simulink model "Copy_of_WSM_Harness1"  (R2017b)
settings: Solver=FixedStepDiscrete  StartTime=0.0  StopTime=2  FixedStep=0.01  RelTol=1e-3  EnableMultiTasking=on
undefined symbols (not defined in the file): sigbuilder_block

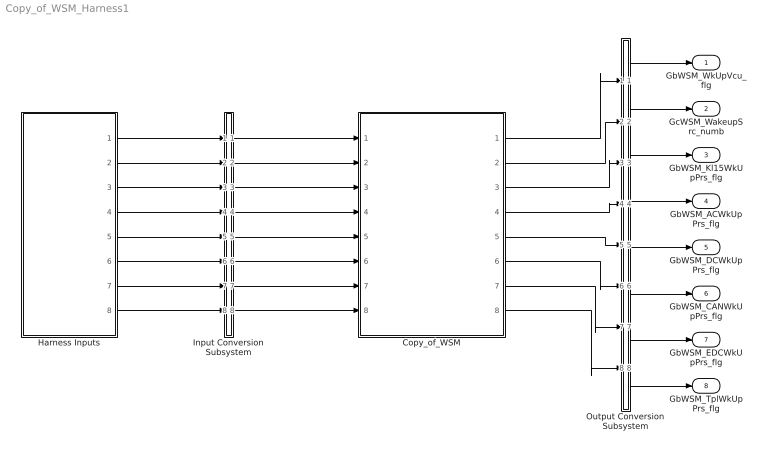
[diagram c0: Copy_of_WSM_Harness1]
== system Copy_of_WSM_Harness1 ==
  Copy_of_WSM : ModelReference  ModelNameDialog=Copy_of_WSM  SimulationMode=Normal  ModelReferenceVersion='M105C102'
  Harness Inputs : Subsystem  Tag=STV Subsys  LoadFcn=sigbuilder_block('load');  StartFcn=sigbuilder_block('start');  StopFcn=sigbuilder_block('stop');  ClipboardFcn=sigbuilder_block('clipboard');  mask(Sigbuilder block){tuvar=[0:10]}
      mask init:
      | if ~strcmp(get_param(bdroot(gcb),'SimulationStatus'),'stopped'),tuvar = sigbuilder_block('maskInit'); end
  Input Conversion Subsystem : Subsystem  Tag=__SLT_ICS__  Description=Signal spec. and routing
  Output Conversion Subsystem : Subsystem  Tag=__SLT_OCS__  Description=Signal spec. and routing
  GbWSM_WkUpVcu_flg : Outport  OutDataTypeStr=boolean  PortDimensions=[1]
  GcWSM_WakeupSrc_numb : Outport  Port=2  OutDataTypeStr=uint16  PortDimensions=[1]
  GbWSM_Kl15WkUpPrs_flg : Outport  Port=3  OutDataTypeStr=boolean  PortDimensions=[1]
  GbWSM_ACWkUpPrs_flg : Outport  Port=4  OutDataTypeStr=boolean  PortDimensions=[1]
  GbWSM_DCWkUpPrs_flg : Outport  Port=5  OutDataTypeStr=boolean  PortDimensions=[1]
  GbWSM_CANWkUpPrs_flg : Outport  Port=6  OutDataTypeStr=boolean  PortDimensions=[1]
  GbWSM_EDCWkUpPrs_flg : Outport  Port=7  OutDataTypeStr=boolean  PortDimensions=[1]
  GbWSM_TplWkUpPrs_flg : Outport  Port=8  OutDataTypeStr=boolean  PortDimensions=[1]
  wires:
  Harness Inputs/1(GbISP_Kl15WkUp_flg) -> Input Conversion Subsystem/1(Inport_1)
  Harness Inputs/2(GbISP_ObcWkUp_flg) -> Input Conversion Subsystem/2(Inport_2)
  Harness Inputs/3(GbLDP_DC12VSply_flg) -> Input Conversion Subsystem/3(Inport_3)
  Harness Inputs/4(GeISP_NetWkUpSt_enum) -> Input Conversion Subsystem/4(Inport_4)
  Harness Inputs/5(GeODP_ObcCcSt_enum) -> Input Conversion Subsystem/5(Inport_5)
  Harness Inputs/6(GbODP_2EBTiout_flg) -> Input Conversion Subsystem/6(Inport_6)
  Harness Inputs/7(GbISP_TFThmRnwyfDet_flg) -> Input Conversion Subsystem/7(Inport_7)
  Harness Inputs/8(GbTRA_TPLRnwyChkFinish_flg) -> Input Conversion Subsystem/8(Inport_8)
  Output Conversion Subsystem/1(Outport_1) -> GbWSM_WkUpVcu_flg/1
  Output Conversion Subsystem/2(Outport_2) -> GcWSM_WakeupSrc_numb/1
  Output Conversion Subsystem/3(Outport_3) -> GbWSM_Kl15WkUpPrs_flg/1
  Output Conversion Subsystem/4(Outport_4) -> GbWSM_ACWkUpPrs_flg/1
  Output Conversion Subsystem/5(Outport_5) -> GbWSM_DCWkUpPrs_flg/1
  Output Conversion Subsystem/6(Outport_6) -> GbWSM_CANWkUpPrs_flg/1
  Output Conversion Subsystem/7(Outport_7) -> GbWSM_EDCWkUpPrs_flg/1
  Output Conversion Subsystem/8(Outport_8) -> GbWSM_TplWkUpPrs_flg/1
  Input Conversion Subsystem/1(Outport_1) -> Copy_of_WSM/1
  Input Conversion Subsystem/2(Outport_2) -> Copy_of_WSM/2
  Input Conversion Subsystem/3(Outport_3) -> Copy_of_WSM/3
  Input Conversion Subsystem/4(Outport_4) -> Copy_of_WSM/4
  Input Conversion Subsystem/5(Outport_5) -> Copy_of_WSM/5
  Input Conversion Subsystem/6(Outport_6) -> Copy_of_WSM/6
  Input Conversion Subsystem/7(Outport_7) -> Copy_of_WSM/7
  Input Conversion Subsystem/8(Outport_8) -> Copy_of_WSM/8
  Copy_of_WSM/1 -> Output Conversion Subsystem/1(Inport_1)
  Copy_of_WSM/2 -> Output Conversion Subsystem/2(Inport_2)
  Copy_of_WSM/3 -> Output Conversion Subsystem/3(Inport_3)
  Copy_of_WSM/4 -> Output Conversion Subsystem/4(Inport_4)
  Copy_of_WSM/5 -> Output Conversion Subsystem/5(Inport_5)
  Copy_of_WSM/6 -> Output Conversion Subsystem/6(Inport_6)
  Copy_of_WSM/7 -> Output Conversion Subsystem/7(Inport_7)
  Copy_of_WSM/8 -> Output Conversion Subsystem/8(Inport_8)

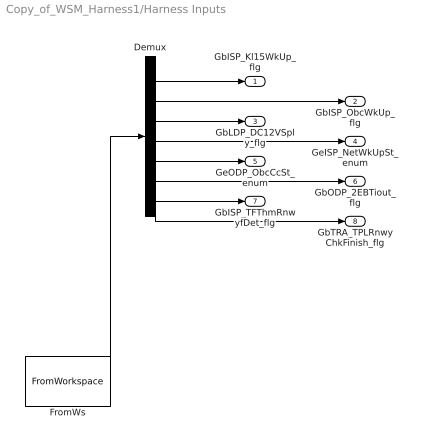
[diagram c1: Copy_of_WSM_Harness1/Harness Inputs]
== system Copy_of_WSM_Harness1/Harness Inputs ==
  Demux : Demux  Tag=STV Demux  Outputs=8
  FromWs : FromWorkspace  Tag=STV FromWs  VariableName=tuvar  SampleTime=0
  GbISP_Kl15WkUp_flg : Outport  Tag=STV Outport
  GbISP_ObcWkUp_flg : Outport  Tag=STV Outport  Port=2
  GbLDP_DC12VSply_flg : Outport  Tag=STV Outport  Port=3
  GeISP_NetWkUpSt_enum : Outport  Tag=STV Outport  Port=4
  GeODP_ObcCcSt_enum : Outport  Tag=STV Outport  Port=5
  GbODP_2EBTiout_flg : Outport  Tag=STV Outport  Port=6
  GbISP_TFThmRnwyfDet_flg : Outport  Tag=STV Outport  Port=7
  GbTRA_TPLRnwyChkFinish_flg : Outport  Tag=STV Outport  Port=8
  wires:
  FromWs/1 -> Demux/1
  Demux/1 -> GbISP_Kl15WkUp_flg/1
  Demux/2 -> GbISP_ObcWkUp_flg/1
  Demux/3 -> GbLDP_DC12VSply_flg/1
  Demux/4 -> GeISP_NetWkUpSt_enum/1
  Demux/5 -> GeODP_ObcCcSt_enum/1
  Demux/6 -> GbODP_2EBTiout_flg/1
  Demux/7 -> GbISP_TFThmRnwyfDet_flg/1
  Demux/8 -> GbTRA_TPLRnwyChkFinish_flg/1

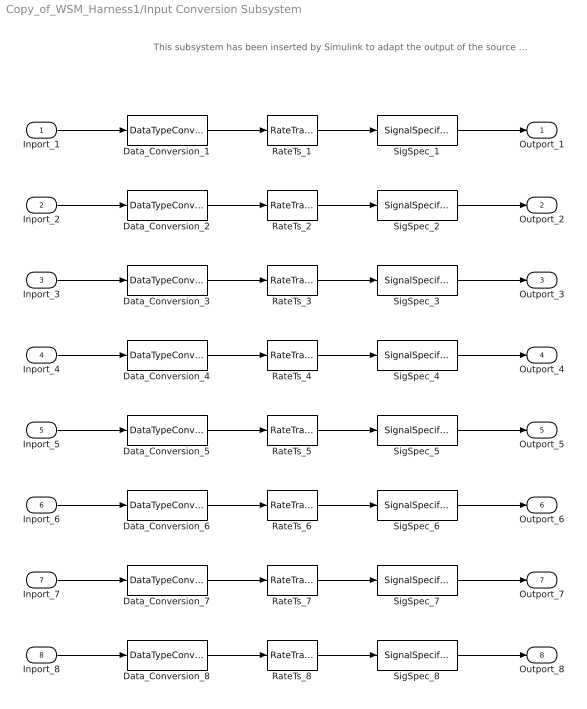
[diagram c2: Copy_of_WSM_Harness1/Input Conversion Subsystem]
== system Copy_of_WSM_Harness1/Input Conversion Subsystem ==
  note: This subsystem has been inserted by Simulink to adapt the output of the source blocks to the interface required by the harnessed component. Modifying the contents of this subsystem may result in compilation and simulation failure.
  Inport_1 : Inport
  Inport_2 : Inport  Port=2
  Inport_3 : Inport  Port=3
  Inport_4 : Inport  Port=4
  Inport_5 : Inport  Port=5
  Inport_6 : Inport  Port=6
  Inport_7 : Inport  Port=7
  Inport_8 : Inport  Port=8
  Data_Conversion_{1..3,6..8} (6 alike) : DataTypeConversion  OutDataTypeStr=boolean
  Data_Conversion_4 : DataTypeConversion  OutDataTypeStr=uint8
  Data_Conversion_5 : DataTypeConversion  OutDataTypeStr=uint8
  RateTs_{1..8} (8 alike) : RateTransition  OutPortSampleTime=0.01
  SigSpec_{1..3,7..8} (5 alike) : SignalSpecification  OutDataTypeStr=boolean  Unit=flag  Dimensions=[1]  SampleTime=0.01
  SigSpec_4 : SignalSpecification  OutDataTypeStr=uint8  Unit=enum  Dimensions=[1]  SampleTime=0.01
  SigSpec_5 : SignalSpecification  OutDataTypeStr=uint8  Unit=numb  Dimensions=[1]  SampleTime=0.01
  SigSpec_6 : SignalSpecification  OutDataTypeStr=boolean  Unit=flg  Dimensions=[1]  SampleTime=0.01
  Outport_1 : Outport
  Outport_2 : Outport  Port=2
  Outport_3 : Outport  Port=3
  Outport_4 : Outport  Port=4
  Outport_5 : Outport  Port=5
  Outport_6 : Outport  Port=6
  Outport_7 : Outport  Port=7
  Outport_8 : Outport  Port=8
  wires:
  SigSpec_1/1 -> Outport_1/1
  RateTs_1/1 -> SigSpec_1/1
  Data_Conversion_1/1 -> RateTs_1/1
  Inport_1/1 -> Data_Conversion_1/1
  SigSpec_2/1 -> Outport_2/1
  RateTs_2/1 -> SigSpec_2/1
  Data_Conversion_2/1 -> RateTs_2/1
  Inport_2/1 -> Data_Conversion_2/1
  SigSpec_3/1 -> Outport_3/1
  RateTs_3/1 -> SigSpec_3/1
  Data_Conversion_3/1 -> RateTs_3/1
  Inport_3/1 -> Data_Conversion_3/1
  SigSpec_4/1 -> Outport_4/1
  RateTs_4/1 -> SigSpec_4/1
  Data_Conversion_4/1 -> RateTs_4/1
  Inport_4/1 -> Data_Conversion_4/1
  SigSpec_5/1 -> Outport_5/1
  RateTs_5/1 -> SigSpec_5/1
  Data_Conversion_5/1 -> RateTs_5/1
  Inport_5/1 -> Data_Conversion_5/1
  SigSpec_6/1 -> Outport_6/1
  RateTs_6/1 -> SigSpec_6/1
  Data_Conversion_6/1 -> RateTs_6/1
  Inport_6/1 -> Data_Conversion_6/1
  SigSpec_7/1 -> Outport_7/1
  RateTs_7/1 -> SigSpec_7/1
  Data_Conversion_7/1 -> RateTs_7/1
  Inport_7/1 -> Data_Conversion_7/1
  SigSpec_8/1 -> Outport_8/1
  RateTs_8/1 -> SigSpec_8/1
  Data_Conversion_8/1 -> RateTs_8/1
  Inport_8/1 -> Data_Conversion_8/1

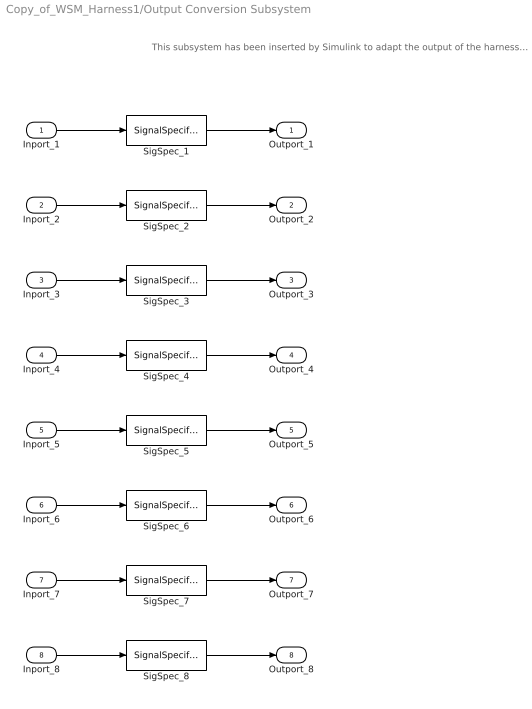
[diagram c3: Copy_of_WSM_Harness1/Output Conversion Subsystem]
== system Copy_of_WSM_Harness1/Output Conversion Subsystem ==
  note: This subsystem has been inserted by Simulink to adapt the output of the harnessed component to the interface required by the sink blocks. Modifying the contents of this subsystem may result in compilation and simulation failure.
  Inport_1 : Inport
  Inport_2 : Inport  Port=2
  Inport_3 : Inport  Port=3
  Inport_4 : Inport  Port=4
  Inport_5 : Inport  Port=5
  Inport_6 : Inport  Port=6
  Inport_7 : Inport  Port=7
  Inport_8 : Inport  Port=8
  SigSpec_{1,3..6,8} (6 alike) : SignalSpecification  OutDataTypeStr=boolean  Unit=flg  Dimensions=[1]  SampleTime=0.01
  SigSpec_2 : SignalSpecification  OutDataTypeStr=uint16  Unit=numb  Dimensions=[1]  SampleTime=0.01
  SigSpec_7 : SignalSpecification  OutDataTypeStr=boolean  Unit=flg  Dimensions=[1]
  Outport_1 : Outport
  Outport_2 : Outport  Port=2
  Outport_3 : Outport  Port=3
  Outport_4 : Outport  Port=4
  Outport_5 : Outport  Port=5
  Outport_6 : Outport  Port=6
  Outport_7 : Outport  Port=7
  Outport_8 : Outport  Port=8
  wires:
  Inport_1/1 -> SigSpec_1/1
  SigSpec_1/1 -> Outport_1/1
  Inport_2/1 -> SigSpec_2/1
  SigSpec_2/1 -> Outport_2/1
  Inport_3/1 -> SigSpec_3/1
  SigSpec_3/1 -> Outport_3/1
  Inport_4/1 -> SigSpec_4/1
  SigSpec_4/1 -> Outport_4/1
  Inport_5/1 -> SigSpec_5/1
  SigSpec_5/1 -> Outport_5/1
  Inport_6/1 -> SigSpec_6/1
  SigSpec_6/1 -> Outport_6/1
  Inport_7/1 -> SigSpec_7/1
  SigSpec_7/1 -> Outport_7/1
  Inport_8/1 -> SigSpec_8/1
  SigSpec_8/1 -> Outport_8/1
